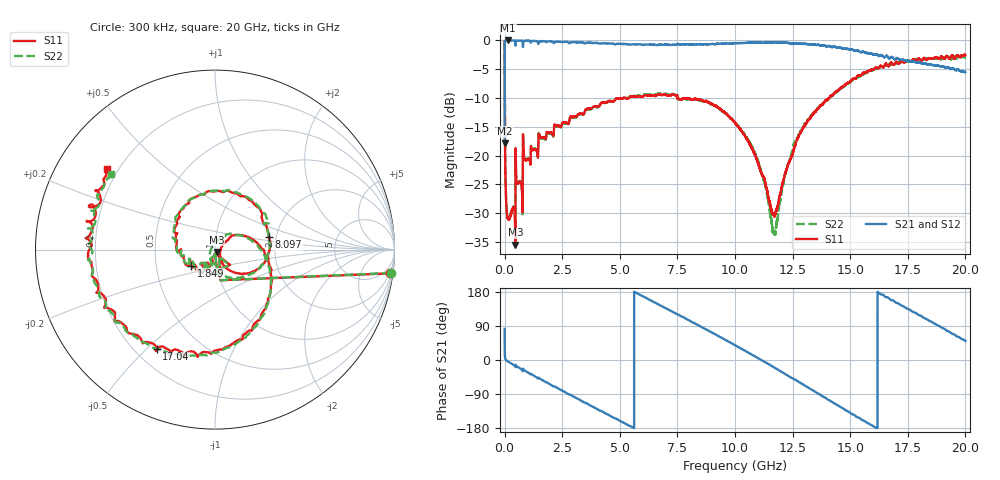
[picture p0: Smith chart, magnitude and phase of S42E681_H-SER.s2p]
!{S42E681}
!Johanson Technology Inc.
!www.johansontechnology.com
!Test Board Conditions:
!Substrate Type  RO4350B
!Substrate Thickness  50 mil
!Substrate Dk  3.66
!TL Type: GCPW
!TL Trace Width  60 mil
!TL Gap  10 mil
!Electrode orientation  Horizontal
!DUT TOPOLOGY	SERIES
!Mounting Pad LxW  14x55 mil
! Created Wed Nov 25 22:25:05 2020
# khz S ma R 50
! 2 Port Network Data from SP1.SP block
! freq  magS11  angS11  magS21  angS21  magS12  angS12  magS22  angS22
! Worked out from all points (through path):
!   20001 points, 300 kHz to 20 GHz, reference 50 ohm
!   highest |S21| = -0.02 dB at 147.3 MHz (marker M1); lowest = -17.9 dB at 300 kHz (marker M2)
!   group delay of S21, straight-line fit = 93.4 ps
!   lowest |S11| = -35.5 dB at 465.3 MHz (marker M3), VSWR 1.03, Z = 51.1 - j1.32 ohm
!   |S11| at or under -10 dB: 7.019 MHz to 5.159 GHz (5.152 GHz wide, 199 % of centre); 5.266 GHz to 5.404 GHz (137.3 MHz wide, 2.57 % of centre); 7.5 GHz to 14.08 GHz (6.584 GHz wide, 61 % of centre)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
!   |S22| runs from -35.7 to -0.1 dB; largest |S21 - S12| = 0.016
!   S11 on the Smith chart (normalised r, x): 300 kHz: 2, -15; 1.849 GHz: 0.76, -0.14; 8.097 GHz: 1.83, +0.28; 17.04 GHz: 0.28, -0.54; 20 GHz: 0.16, +0.32
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300  0.9862 -7.7  0.1277 82.1  0.1271 81.9  0.9881 -7.6
102300  0.0312 -88.3  0.9975 -2.1  0.9966 -2.1  0.03179 -88.4
147300  0.02847 -89.8  0.9976 -4.0  0.9974 -4.0  0.02884 -90.4
465300  0.01688 -50.0  0.984 -17.3  0.9851 -17.2  0.01639 -55.0
890300  0.09177 -116.7  0.9908 -28.5  0.9906 -28.5  0.09257 -119.4
1849300  0.1596 -145.9  0.9758 -59.6  0.9761 -59.6  0.157 -153.2
3334300  0.2306 158.0  0.9602 -107.8  0.9604 -107.8  0.227 165.9
5054300  0.3129 109.1  0.9309 -162.2  0.931 -162.2  0.3119 110.1
6667300  0.3389 60.8  0.9125 147.4  0.9118 147.3  0.3443 57.1
8097300  0.3084 13.0  0.9219 101.4  0.9216 101.4  0.3054 10.3
8992300  0.2805 -16.6  0.9302 72.5  0.9297 72.6  0.2783 -17.4
1.00003e7  0.1938 -44.3  0.9438 39.1  0.9433 39.2  0.1943 -55.2
1.09363e7  0.09376 -61.2  0.957 7.1  0.9572 7.1  0.09635 -98.6
1.17003e7  0.02998 -9.5  0.9583 -19.6  0.9595 -19.6  0.02198 158.0
1.25603e7  0.1148 40.0  0.9363 -50.2  0.9356 -50.1  0.1279 44.3
1.33343e7  0.2213 13.4  0.9223 -78.6  0.9217 -78.6  0.2251 9.3
1.40793e7  0.3152 -16.3  0.8954 -106.0  0.8944 -105.6  0.3187 -18.2
1.50373e7  0.4456 -54.7  0.8275 -141.2  0.8304 -141.1  0.439 -50.9
1.66673e7  0.5976 -109.7  0.7059 163.7  0.7094 162.9  0.6133 -106.0
1.70393e7  0.6427 -120.4  0.7 150.4  0.691 150.8  0.634 -118.8
1.85623e7  0.6917 -171.8  0.6097 99.4  0.6069 99.3  0.6947 -166.5
2e7  0.7457 143.2  0.5305 50.4  0.5313 50.8  0.7218 143.6
